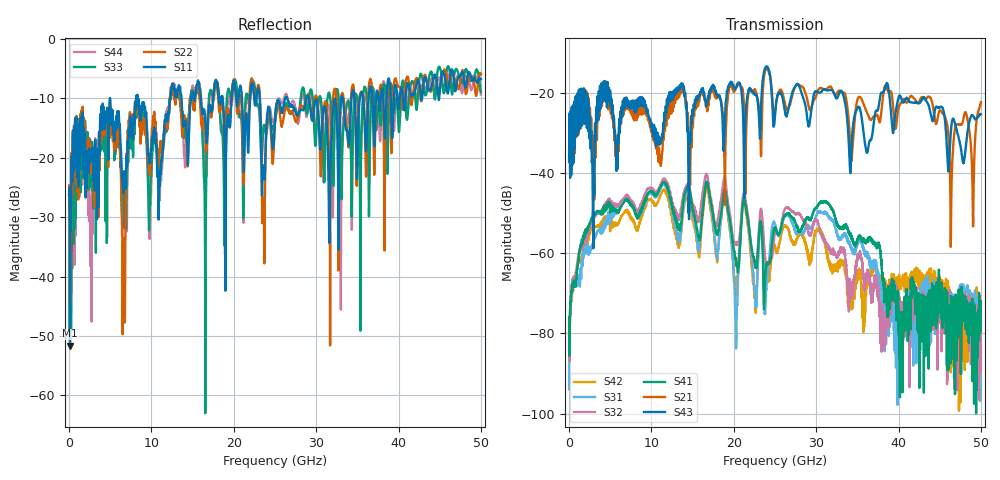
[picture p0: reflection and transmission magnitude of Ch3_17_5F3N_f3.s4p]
!Agilent Technologies,N5247A,US51170199,A.09.90.13
!Agilent N5247A: A.09.90.13
!Date: Wednesday, December 09, 2015 09:20:01
!Correction: S11(Full 4 Port(1,2,3,4))
!S12(Full 4 Port(1,2,3,4))
!S13(Full 4 Port(1,2,3,4))
!S14(Full 4 Port(1,2,3,4))
!S21(Full 4 Port(1,2,3,4))
!S22(Full 4 Port(1,2,3,4))
!S23(Full 4 Port(1,2,3,4))
!S24(Full 4 Port(1,2,3,4))
!S31(Full 4 Port(1,2,3,4))
!S32(Full 4 Port(1,2,3,4))
!S33(Full 4 Port(1,2,3,4))
!S34(Full 4 Port(1,2,3,4))
!S41(Full 4 Port(1,2,3,4))
!S42(Full 4 Port(1,2,3,4))
!S43(Full 4 Port(1,2,3,4))
!S44(Full 4 Port(1,2,3,4))
!S4P File: Measurements: <S11,S12,S13,S14>,
!<S21,S22,S23,S24>,
!<S31,S32,S33,S34>,
!<S41,S42,S43,S44>:
# Hz S  dB  R 50
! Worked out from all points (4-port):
!   3201 points, 10 MHz to 50 GHz, reference 50 ohm
!   strongest paths, dB at 10 MHz, 12.51 GHz, 25 GHz, 37.5 GHz, 50 GHz:
!     S43: -37.1, -19.8, -25.4, -24.2, -25.3
!     S21: -37.2, -22.6, -24.8, -25.9, -22.3
!     S41: -76.0, -48.5, -53.6, -57.6, -72.0
!     S32: -79.8, -47.7, -55.0, -69.8, -79.2
!     S31: -93.9, -49.6, -52.6, -66.8, -83.8
!     S42: -78.6, -51.8, -58.3, -66.5, -75.5
!   lowest |S11| = -51.6 dB at 119.4 MHz (marker M1), VSWR 1.01, Z = 50.1 + j0.253 ohm
!   |S11| at or under -10 dB: start of sweep to 4.962 GHz; 8.344 GHz to 12.3 GHz (3.959 GHz wide, 38.3 % of centre); 29.14 GHz to 33.05 GHz (3.907 GHz wide, 12.6 % of centre)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
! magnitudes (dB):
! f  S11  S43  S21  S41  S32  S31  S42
! 10 MHz  -26.4  -37.1  -37.2  -76.0  -79.8  -93.9  -78.6
! 119.4 MHz  -51.6  -36.9  -36.2  -75.1  -74.0  -75.8  -77.0
! 16.68 GHz  -17.2  -22.8  -23.3  -42.3  -40.2  -41.9  -43.6
! 20.24 GHz  -9.0  -18.8  -18.6  -61.2  -57.3  -75.9  -69.5
! 21.29 GHz  -18.6  -41.0  -25.8  -46.6  -45.1  -46.2  -47.3
! 22.57 GHz  -11.1  -20.3  -19.0  -62.0  -62.1  -69.7  -70.6
! 50 GHz  -6.8  -25.3  -22.3  -72.0  -79.2  -83.8  -75.5
